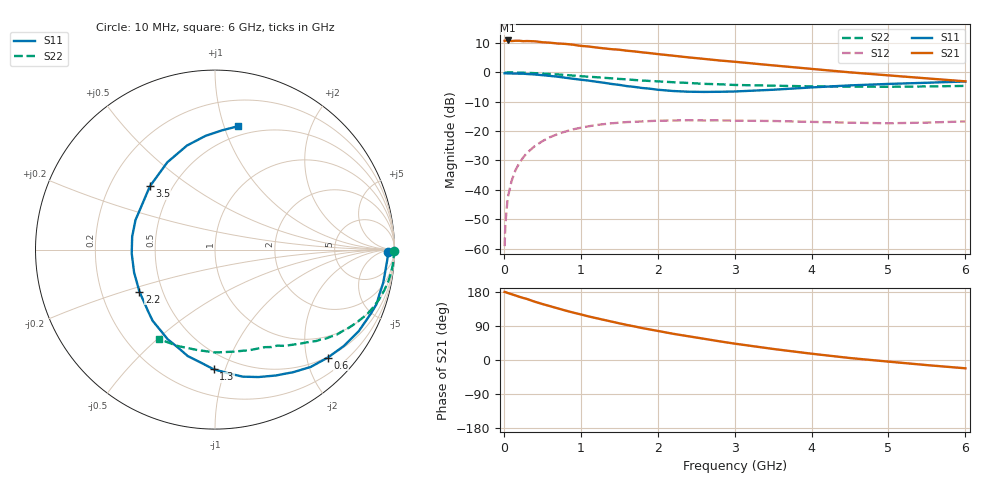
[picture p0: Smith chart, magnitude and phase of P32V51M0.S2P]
! SIEMENS Small Signal Semiconductors
! BFP181
! Si NPN RF Bipolar Junction Transistor in SOT143
! VCE = 2.5 V  IC = 1 mA
! Common Emitter S-Parameters:  March  1996
# GHz  S  MA  R  50
!  f  S11  S21  S12  S22
! GHz  MAG  ANG  MAG  ANG  MAG  ANG  MAG  ANG
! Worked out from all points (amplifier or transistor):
!   36 points, 10 MHz to 6 GHz, reference 50 ohm
!   highest |S21| = 10.9 dB at 50 MHz (marker M1)
!   |S21| within 3 dB of that: start of sweep to 1.416 GHz
!   unconditionally stable (mu >= 1): 3.067 GHz to end of sweep
!   at 250 MHz: K = 0.09, MSG = 19.8 dB, |S12| = -29.0 dB
!   at 1.4 GHz: K = 0.50, MSG = 12.6 dB, |S12| = -17.3 dB
!   at 6 GHz: K = 1.29, MAG = 3.6 dB, |S12| = -16.7 dB
!   lowest NFmin = 1.30 dB at 450 MHz
!   S11 on the Smith chart (normalised r, x): 10 MHz: 47, -20; 600 MHz: 0.49, -2.41; 1.3 GHz: 0.38, -0.91; 2.2 GHz: 0.37, -0.23; 3.5 GHz: 0.38, +0.36; 6 GHz: 0.41, +1.12
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0.01  0.9646 -0.9  3.444 179.6  0.0011 90.6  0.9992 -0.3
0.02  0.9639 -1.7  3.464 179.3  0.0026 88.5  0.9899 -0.7
0.05  0.9615 -3.4  3.493 176.9  0.0073 90.6  0.9966 -1.8
0.1  0.9562 -7.4  3.41 173.7  0.0141 84.7  0.9955 -3.4
0.15  0.9552 -11.2  3.455 170.4  0.0215 81.8  0.994 -5.2
0.25  0.9501 -18.6  3.395 163.8  0.0354 77.8  0.9863 -8.6
0.3  0.9389 -22.3  3.412 161.1  0.0424 75.5  0.982 -10.3
0.4  0.9209 -29.6  3.381 154.0  0.0553 70.7  0.9697 -13.6
0.6  0.8702 -43.7  3.198 142.1  0.0788 61.4  0.9397 -19.8
0.8  0.81 -57.5  3.051 130.6  0.0983 53.2  0.903 -25.2
0.9  0.7786 -64.3  2.957 125.2  0.1071 49.2  0.8823 -27.9
1.1  0.7245 -77.7  2.758 115.1  0.1207 42.3  0.8431 -32.6
1.3  0.6664 -90.7  2.564 105.9  0.1314 35.9  0.8083 -36.8
1.5  0.6125 -104.3  2.429 96.8  0.139 30.5  0.7732 -40.4
1.8  0.5417 -124.4  2.19 84.2  0.1462 23.8  0.7266 -45.3
2.2  0.4816 -151.0  1.922 69.2  0.1516 16.1  0.6797 -51.4
2.8  0.4671 171.1  1.595 49.4  0.1524 7.6  0.6269 -60.0
3.5  0.506 135.8  1.314 29.2  0.1487 1.6  0.5932 -70.7
4  0.5544 118.6  1.146 16.6  0.1436 -1.2  0.5778 -79.8
4.5  0.6003 105.1  1.001 5.2  0.1391 -2.7  0.5732 -90.0
5.5  0.6657 86.6  0.79 -13.5  0.1396 0.5  0.5759 -111.3
6  0.6998 79.3  0.703 -21.9  0.1462 1.3  0.5886 -122.3
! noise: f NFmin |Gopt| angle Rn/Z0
0.45  1.3  0.7  18  0.5
0.9  1.4  0.6  39  0.52
1.8  1.85  0.4  81  0.47
